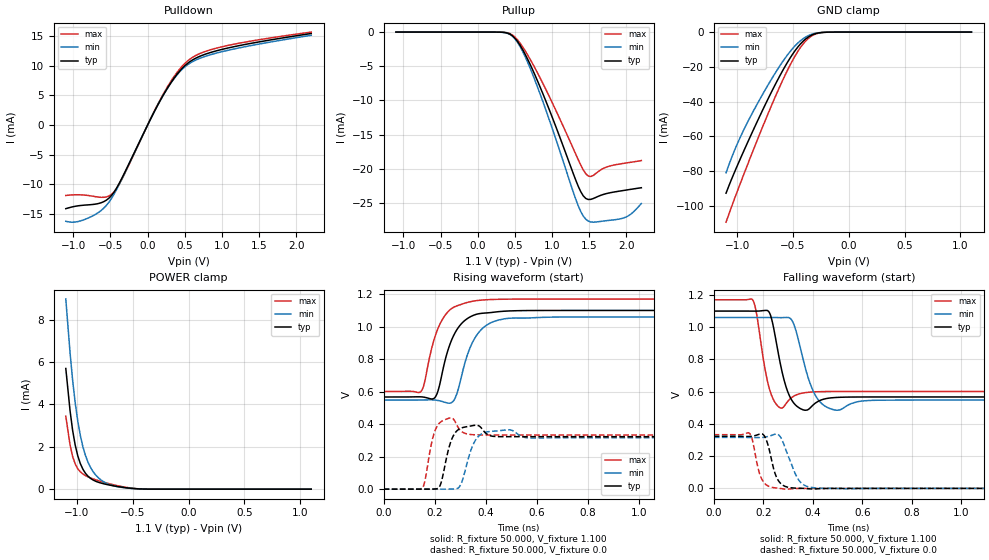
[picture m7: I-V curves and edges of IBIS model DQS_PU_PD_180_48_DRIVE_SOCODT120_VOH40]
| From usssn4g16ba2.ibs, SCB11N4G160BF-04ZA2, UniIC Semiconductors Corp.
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|   Model DQS_PU_PD_180_48_DRIVE_SOCODT120_VOH40
[Model] DQS_PU_PD_180_48_DRIVE_SOCODT120_VOH40
Model_type I/O
Polarity   Inverting
Vinl =  0.135V
Vinh =  0.305V
Vmeas =  0.220V
Rref =  50.000
Vref =  0.220V
C_comp   1.020pF   1.010pF   1.030pF
[Model Spec]
Vinh   0.305V   0.297V   0.319V
Vinl   0.135V   0.127V   0.149V
Vmeas   0.220V   0.212V   0.234V
Vref   0.220V   0.212V   0.234V
Rref   50.000   NA   NA
[Temperature Range]   25.000   0.105k   -40.000
[Voltage Range]   1.100V   1.060V   1.170V
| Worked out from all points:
|   slope of the pulldown table from 0 to 0.165 V, typ, clamps not added: 41 ohm
|   GND clamp passes 1 mA (typ) near -0.30 V on its own axis
|   POWER clamp passes 1 mA (typ) near -0.95 V on its own axis
|   rising waveform, R_fixture 50.000, V_fixture 1.100: 20-80 % time 68ps typ, 70.8ps min, 66.8ps max; typ from 0.567 V to 1.1 V
|   rising waveform, R_fixture 50.000, V_fixture 0.0: 20-80 % time 27.2ps typ, 34.6ps min, 21.7ps max; typ from 0 V to 0.323 V
|   falling waveform, R_fixture 50.000, V_fixture 1.100: 20-80 % time 41.7ps typ, 53.6ps min, 34.3ps max; typ from 1.1 V to 0.567 V
|   falling waveform, R_fixture 50.000, V_fixture 0.0: 20-80 % time 34ps typ, 50.4ps min, 30.5ps max; typ from 0.323 V to 0 V
[Pulldown]
|Voltage   I(typ)   I(min)   I(max)
-1.1V     -14.07mA   -16.18mA   -11.85mA
-930mV    -13.58mA   -16.22mA   -11.73mA
-726mV    -13.35mA   -15.21mA   -12mA
-556mV    -12.65mA   -13.54mA   -12.1mA
-454mV    -11.34mA   -11.69mA   -11.29mA
-318mV    -8.242mA   -8.339mA   -8.422mA
192mV     4.628mA    4.609mA    4.791mA
362mV     7.992mA    7.909mA    8.275mA
532mV     10.32mA    10.1mA     10.72mA
702mV     11.57mA    11.22mA    12.02mA
1.008V    12.75mA    12.37mA    13.19mA
2.2V      15.4mA     15.1mA     15.64mA
[Pullup]
|Voltage   I(typ)   I(min)   I(max)
-1.1V     1.8nA      19.34nA    0A
432mV     -294.2uA   -340.2uA   -214.5uA
568mV     -1.899mA   -2.087mA   -1.603mA
738mV     -5.508mA   -6.173mA   -4.628mA
976mV     -11.74mA   -13.27mA   -9.734mA
1.316V    -21.59mA   -24.38mA   -17.8mA
1.418V    -23.93mA   -26.88mA   -20.13mA
1.52V     -24.46mA   -27.76mA   -21.11mA
1.724V    -23.63mA   -27.58mA   -19.76mA
1.928V    -23.21mA   -27.28mA   -19.25mA
2.064V    -22.98mA   -26.57mA   -19.02mA
2.2V      -22.76mA   -25.06mA   -18.79mA
[GND_clamp]
|Voltage   I(typ)   I(min)   I(max)
-1.1V     -92.78mA   -81.05mA   -109.5mA
-1.031V   -81.73mA   -69.22mA   -97.17mA
-939mV    -68.18mA   -56.02mA   -81.64mA
-824mV    -52mA      -41.83mA   -62.83mA
-686mV    -33.62mA   -26.41mA   -41.32mA
-571mV    -19.76mA   -15.06mA   -24.85mA
-479mV    -10.5mA    -7.76mA    -13.5mA
-410mV    -5.313mA   -3.84mA    -6.916mA
-341mV    -2.007mA   -1.45mA    -2.59mA
-272mV    -506.9uA   -403.5uA   -609.8uA
-180mV    -45.65uA   -51.35uA   -43.55uA
1.1V      0A         0A         0A
[POWER_clamp]
|Voltage   I(typ)   I(min)   I(max)
-1.1V     5.691mA    8.967mA    3.44mA
-1.062V   3.709mA    6.444mA    2.092mA
-1.039V   2.781mA    5.152mA    1.546mA
-1.016V   2.086mA    4.085mA    1.193mA
-970mV    1.21mA     2.539mA    818.5uA
-947mV    943.7uA    2.005mA    716.7uA
-901mV    610.1uA    1.27mA     581.3uA
-855mV    430.7uA    824.1uA    484.6uA
-786mV    289.9uA    439.4uA    366uA
-671mV    155.9uA    155.9uA    203.6uA
-441mV    13.2uA     12.79uA    15.03uA
1.1V      0A         0A         0A
[Ramp]
| variable   typ   min   max
dV/dt_r   0.194/27.321p   0.190/34.549p   0.200/21.820p
dV/dt_f   0.320/41.913p   0.307/53.687p   0.341/34.362p
R_load = 50.000
[Rising Waveform]
R_fixture= 50.000
V_fixture= 1.100
V_fixture_min= 1.060
V_fixture_max= 1.170
|time   V(typ)   V(min)   V(max)
0s        567.3mV    548.1mV    601.6mV
146ps     568.2mV    548.7mV    600.9mV
203ps     569mV      548.1mV    948.8mV
267ps     922.3mV    534.4mV    1.113V
286ps     980.6mV    585.7mV    1.128V
333ps     1.056V     850.8mV    1.152V
369ps     1.079V     958.7mV    1.161V
420ps     1.087V     1.025V     1.167V
504ps     1.098V     1.053V     1.17V
3ns       1.1V       1.06V      1.17V
[Rising Waveform]
R_fixture= 50.000
V_fixture= 0.0
V_fixture_min= 0.0
V_fixture_max= 0.0
|time   V(typ)   V(min)   V(max)
0s        2.854uV    10.37uV    663.5nV
151ps     13.23uV    43.86uV    6.41mV
191ps     550.8uV    56.09uV    308.7mV
218ps     14.08mV    179uV      406.2mV
263ps     294mV      359.6uV    439.2mV
302ps     375.2mV    29.31mV    358.9mV
366ps     393.5mV    317.3mV    334.1mV
481ps     322.9mV    364.8mV    333.3mV
570ps     323.1mV    315.1mV    333.3mV
3ns       323.1mV    316.4mV    333.3mV
[Falling Waveform]
R_fixture= 50.000
V_fixture= 1.100
V_fixture_min= 1.060
V_fixture_max= 1.170
|time   V(typ)   V(min)   V(max)
0s        1.1V       1.06V      1.17V
159ps     1.1V       1.06V      1.165V
225ps     1.089V     1.06V      615.5mV
272ps     749.5mV    1.059V     497.8mV
314ps     549.7mV    1.046V     563.1mV
347ps     497.4mV    887.9mV    587.3mV
411ps     530.1mV    575.4mV    599.3mV
495ps     564.3mV    485.2mV    601.4mV
670ps     567.3mV    547.3mV    601.6mV
3ns       567.3mV    548.1mV    601.6mV
[Falling Waveform]
R_fixture= 50.000
V_fixture= 0.0
V_fixture_min= 0.0
V_fixture_max= 0.0
|time   V(typ)   V(min)   V(max)
0s        323.1mV    316.4mV    333.3mV
144ps     322.3mV    315.9mV    342.1mV
182ps     335.3mV    315.3mV    106.9mV
199ps     334.8mV    316.6mV    44.37mV
217ps     279.1mV    321.6mV    16.87mV
252ps     74.08mV    337.1mV    2.862mV
290ps     11.51mV    244mV      -4.594mV
343ps     1.112mV    51.66mV    -606uV
413ps     -2.954mV   2.692mV    -14.98uV
3ns       -992nV     10.13uV    -2.425uV
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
